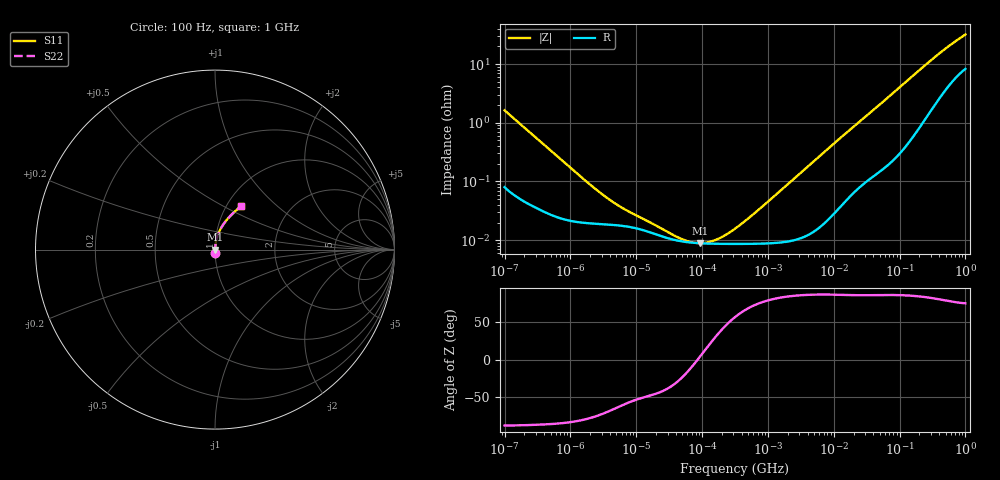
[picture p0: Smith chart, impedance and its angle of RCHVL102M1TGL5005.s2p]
! RCHVL102M1TGL5005  S-PARAMETER MODEL  (AEC-Q200 qualified)
! Model Generated by ELNA Corporation (http://www.ty-top.com)
! Version 1.0
! ELNA Control No. 231123
! Copyright (c) 2023 ELNA CO.,LTD. All Rights Reserved.
! Products Name : CONDUCTIVE POLYMER HYBRID ALUMINUM ELECTROLYTIC CAPACITORS
! Characteristics :
!  Capacitance  :  1000uF  ,  Rated voltage  :  25V
!  Operating Temp. Range  :  -55 to +125  ,  Endurance  :  8000hr at 125
!  Dimension ÓD  :  12.5mm  ,  Dimension L  :  13.5mm
! Frequency Range : 100Hz - 1GHz
! External Node Assignments :
!  1  o---| |---o  2
# MHz S RI R 50
!Freq[MHz].  S11 Real  S11 Imag  S21 Real  S21 Imag  S12 Real  S12 Imag  S22 Real  S22 Imag
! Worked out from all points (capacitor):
!   401 points, 100 Hz to 1 GHz, reference 50 ohm
!   read as one part in series: C = 974 uF near 108 Hz
!   lowest |Z| = 8.91 mohm at 94.41 kHz (marker M1)
!   series resonance near 85.38 kHz, so ESL is about 3.6 nH
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0.0001  0.00106 -0.0163  0.9989 0.0163  0.9989 0.0163  0.00106 -0.0163
0.000113  0.000916 -0.0144  0.9991 0.0144  0.9991 0.0144  0.000916 -0.0144
0.001488  0.000201 -0.00115  0.9998 0.00115  0.9998 0.00115  0.000201 -0.00115
0.002951  0.000188 -0.000592  0.9998 0.000592  0.9998 0.000592  0.000188 -0.000592
0.004983  0.00018 -0.000367  0.9998 0.000367  0.9998 0.000367  0.00018 -0.000367
0.007762  0.000169 -0.000255  0.9998 0.000255  0.9998 0.000255  0.000169 -0.000255
0.022131  0.000121 -0.000115  0.9999 0.000115  0.9999 0.000115  0.000121 -0.000115
0.037368  0.000102 -6.54e-05  0.9999 6.54e-05  0.9999 6.54e-05  0.000102 -6.54e-05
0.051582  9.48e-05 -3.85e-05  0.9999 3.85e-05  0.9999 3.85e-05  9.48e-05 -3.85e-05
0.05821  9.3e-05 -2.9e-05  0.9999 2.9e-05  0.9999 2.9e-05  9.3e-05 -2.9e-05
0.094406  8.88e-05 7.61e-06  0.9999 -7.61e-06  0.9999 -7.61e-06  8.88e-05 7.61e-06
0.147062  8.72e-05 4.34e-05  0.9999 -4.34e-05  0.9999 -4.34e-05  8.72e-05 4.34e-05
0.165959  8.7e-05 5.44e-05  0.9999 -5.44e-05  0.9999 -5.44e-05  8.7e-05 5.44e-05
0.220039  8.66e-05 8.35e-05  0.9999 -8.35e-05  0.9999 -8.35e-05  8.66e-05 8.35e-05
0.316228  8.65e-05 0.000131  0.9999 -0.000131  0.9999 -0.000131  8.65e-05 0.000131
0.737055  8.73e-05 0.000325  0.9999 -0.000325  0.9999 -0.000325  8.73e-05 0.000325
4.704354  0.000139 0.0021  0.9999 -0.0021  0.9999 -0.0021  0.000139 0.0021
69.9842  0.00278 0.0281  0.9972 -0.0281  0.9972 -0.0281  0.00278 0.0281
169.8244  0.0106 0.0659  0.9894 -0.0659  0.9894 -0.0659  0.0106 0.0659
365.1741  0.0391 0.1291  0.9609 -0.1291  0.9609 -0.1291  0.0391 0.1291
641.9482  0.0888 0.1911  0.9112 -0.1911  0.9112 -0.1911  0.0888 0.1911
1000  0.1456 0.243  0.8544 -0.243  0.8544 -0.243  0.1456 0.243
